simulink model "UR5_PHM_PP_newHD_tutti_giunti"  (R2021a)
settings: Solver=ode14x  StartTime=0.0  StopTime=Sim.time  FixedStep=Sim.dt  MaxStep=Sim.dt  RelTol=1e-3  EnableMultiTasking=on
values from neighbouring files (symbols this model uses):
  alpha_n = 0.98*pi/180    (= 0.0171042266695)    [parameters.m]
  alpha_t = 30*pi/180    (= 0.523598775598)    [parameters.m]
  alpha_TTS = 0    [parameters.m]
  alpha_Tw_L = -6.9e-4    (= -0.00069)    [parameters.m]
  alpha_Tw_R = 3.9e-3    (= 0.0039)    [parameters.m]
  Beta_TTS = 0    [parameters.m]
  c1 = 1e-2    (= 0.01)    [parameters.m]
  c2 = 1e-2    (= 0.01)    [parameters.m]
  c3 = 1e-2    (= 0.01)    [parameters.m]
  c4 = 1e-2    (= 0.01)    [parameters.m]
  c5 = 1e-2    (= 0.01)    [parameters.m]
  c6 = 1e-2    (= 0.01)    [parameters.m]
  Cb1 = 1.8e3    (= 1800)    [parameters.m]
  Cb2 = 1.8e3    (= 1800)    [parameters.m]
  Cb3 = 1.8e3    (= 1800)    [parameters.m]
  Cb4 = 1.8e3    (= 1800)    [parameters.m]
  Cb5 = 1.8e3    (= 1800)    [parameters.m]
  Cb6 = 1.8e3    (= 1800)    [parameters.m]
  Cth_housing = 153.90    (= 153.9)    [parameters.m]
  Cth_w = 74.20    (= 74.2)    [parameters.m]
  dt_PP = 0.05    [parameters.m]
  Fric1 = [fc_1/2 1e1 fc_1 fv_1]    [parameters.m]
  Fric2 = [fc_2/2 1e1 fc_2 fv_2]    [parameters.m]
  Fric3 = [fc_3/2 1e1 fc_3 fv_3]    [parameters.m]
  Fric4 = [fc_4/2 1e1 fc_4 fv_4]    [parameters.m]
  Fric5 = [fc_5/2 1e1 fc_5 fv_5]    [parameters.m]
  Fric6 = [fc_6/2 1e1 fc_6 fv_6]    [parameters.m]
  Hth_housing = 0.30    (= 0.3)    [parameters.m]
  Hth_w = 1.14    [parameters.m]
  I_actual = I_actual(1:10,:)    [trajcutting.m]
  J_CS1 = 7.12e-5    (= 7.12e-05)    [parameters.m]
  J_CS2 = 7.12e-5    (= 7.12e-05)    [parameters.m]
  J_CS3 = 7.12e-5    (= 7.12e-05)    [parameters.m]
  J_CS4 = 6e-6    (= 6e-06)    [parameters.m]
  J_CS5 = 6e-6    (= 6e-06)    [parameters.m]
  J_CS6 = 6e-6    (= 6e-06)    [parameters.m]
  J_FS1 = 1.62e-7    (= 1.62e-07)    [parameters.m]
  J_FS2 = 1.62e-7    (= 1.62e-07)    [parameters.m]
  J_FS3 = 1.62e-7    (= 1.62e-07)    [parameters.m]
  J_FS4 = 4.97e-8    (= 4.97e-08)    [parameters.m]
  J_FS5 = 4.97e-8    (= 4.97e-08)    [parameters.m]
  J_FS6 = 4.97e-8    (= 4.97e-08)    [parameters.m]
  J_WG1 = 3.56e-5    (= 3.56e-05)    [parameters.m]
  J_WG2 = 3.56e-5    (= 3.56e-05)    [parameters.m]
  J_WG3 = 3.56e-5    (= 3.56e-05)    [parameters.m]
  J_WG4 = 3e-6    (= 3e-06)    [parameters.m]
  J_WG5 = 3e-6    (= 3e-06)    [parameters.m]
  J_WG6 = 3e-6    (= 3e-06)    [parameters.m]
  K_i = 1    [parameters.m]
  K_p = 1    [parameters.m]
  K_torsCS1 = 4.78e6    (= 4780000)    [parameters.m]
  K_torsCS2 = 4.78e6    (= 4780000)    [parameters.m]
  K_torsCS3 = 4.78e6    (= 4780000)    [parameters.m]
  K_torsCS4 = 1.06e6    (= 1060000)    [parameters.m]
  K_torsCS5 = 1.06e6    (= 1060000)    [parameters.m]
  K_torsCS6 = 1.06e6    (= 1060000)    [parameters.m]
  K_torsWG1 = 9.56e5    (= 956000)    [parameters.m]
  K_torsWG2 = 9.56e5    (= 956000)    [parameters.m]
  K_torsWG3 = 9.56e5    (= 956000)    [parameters.m]
  K_torsWG4 = 1.84e5    (= 184000)    [parameters.m]
  K_torsWG5 = 1.84e5    (= 184000)    [parameters.m]
  K_torsWG6 = 1.84e5    (= 184000)    [parameters.m]
  K_v = 1    [parameters.m]
  Kb1 = 0.51e8    (= 51000000)    [parameters.m]
  Kb2 = 0.51e8    (= 51000000)    [parameters.m]
  Kb3 = 0.51e8    (= 51000000)    [parameters.m]
  Kb4 = 1.98e7    (= 19800000)    [parameters.m]
  Kb5 = 1.98e7    (= 19800000)    [parameters.m]
  Kb6 = 1.98e7    (= 19800000)    [parameters.m]
  Km1 = 1.2e9    (= 1200000000)    [parameters.m]
  Km2 = 1.2e9    (= 1200000000)    [parameters.m]
  Km3 = 1.2e9    (= 1200000000)    [parameters.m]
  Km4 = 5.55e8    (= 555000000)    [parameters.m]
  Km5 = 5.55e8    (= 555000000)    [parameters.m]
  Km6 = 5.55e8    (= 555000000)    [parameters.m]
  Kt1 = 0.96e5    (= 96000)    [parameters.m]
  Kt2 = 0.96e5    (= 96000)    [parameters.m]
  Kt3 = 0.96e5    (= 96000)    [parameters.m]
  Kt4 = 1.15e4    (= 11500)    [parameters.m]
  Kt5 = 1.15e4    (= 11500)    [parameters.m]
  Kt6 = 1.15e4    (= 11500)    [parameters.m]
  L = Motor.L_2/2    [parameters.m]
  m2 = polyfit(Temp(:,2),pBn_UR5_f_Temp(:,2),1)    [parameters.m]
  mb2 = polyfit(Temp(:,8),pBn_UR5_f_Temp(:,8),1)    [parameters.m]
  pickTime = t_pick(traj)    [parameters.m]
  placeTime = t_place(traj)    [parameters.m]
  q0 = q_target(1,:)    [testlaw_PP.m]
  q_CS01 = x(6)    [parameters.m]
  q_CS02 = x(6)    [parameters.m]
  q_CS03 = x(6)    [parameters.m]
  q_CS04 = x(6)    [parameters.m]
  q_CS05 = x(6)    [parameters.m]
  q_CS06 = x(6)    [parameters.m]
  q_WG01 = x(1)    [parameters.m]
  q_WG02 = x(1)    [parameters.m]
  q_WG03 = x(1)    [parameters.m]
  q_WG04 = x(1)    [parameters.m]
  q_WG05 = x(1)    [parameters.m]
  q_WG06 = x(1)    [parameters.m]
  quant_i = [Motor.imax1 Motor.imax2      Motor.imax3 Motor.imax4 Motor.imax5 Motor.imax6]/2^16    [parameters.m]
  R = Motor.R_2/2    [parameters.m]
  rg1 = 0.028    [parameters.m]
  rg2 = 0.028    [parameters.m]
  rg3 = 0.028    [parameters.m]
  rg4 = 0.0155    [parameters.m]
  rg5 = 0.0155    [parameters.m]
  rg6 = 0.0155    [parameters.m]
  sigma_p = 444.29    [parameters.m]
  sigma_v = 2*pi*1000    (= 6283.18530718)    [parameters.m]
  stiff_red = 1    [parameters.m]
  T_0 = Sim.temp    [parameters.m]
  T_switch = 1e-4    (= 0.0001)    [parameters.m]
  tau_i = 1/(fc_i*2*pi)    (= 7.95774715459e-05)    [parameters.m]
  U_s = 48    [parameters.m]
  var_i = 1e-1*[.0167 .0184 .0144 .0016      .0011 .0007]    [parameters.m]
  var_p = 1e-6*[.0943 .3877      .3478 .5436 .3400 .2081]    [parameters.m]
  var_v = 1e-4*[.0738 .1452      .1564 .4623 .1824 .0917]    [parameters.m]
  Wf_TTS_0 = 0    [parameters.m]
  Wf_TTS_ONOFF = 0    [parameters.m]
  x2_01 = x(3)    [parameters.m]
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undefined symbols (not defined in the file or in its folder): deg, Driver1, Driver2, Driver3, Driver4, Driver5, Driver6, elseif, geom, Ground, J1, J2, J3, J4, J5, J6, kg, L1, L2, L3, L4, L5, L6, LINK0, LINK1, LINK2, LINK3, LINK4, LINK5, LINK6, m, Motor, N, payload, ROBOTIQ_FT, s, Sim, Tool, X, Y, Z
libraries: sm_lib x35, nesl_utility x30, simulink x23, simulink_extras x11, spsTriangleGeneratorLib x6
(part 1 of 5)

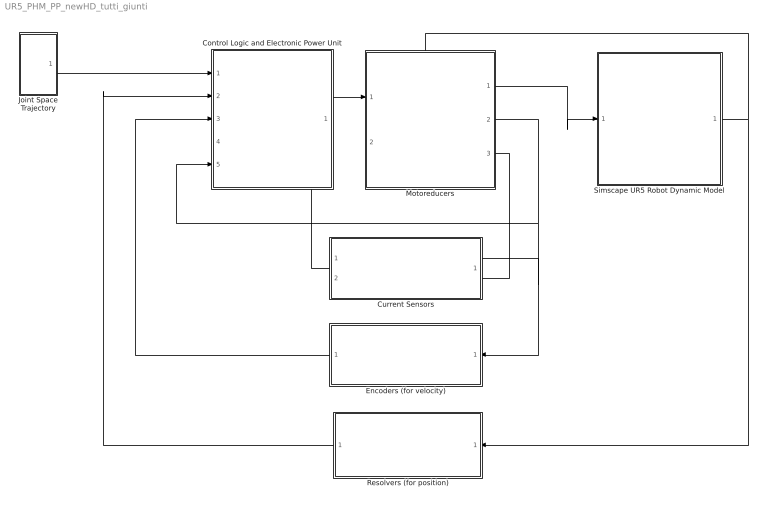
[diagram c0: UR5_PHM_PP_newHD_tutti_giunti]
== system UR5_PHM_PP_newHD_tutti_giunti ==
  Control Logic and Electronic Power Unit : Subsystem
  Current Sensors : Subsystem
  Encoders (for velocity) : Subsystem
  Joint Space Trajectory : Subsystem
  Motoreducers : Subsystem
  Resolvers (for position) : Subsystem
  Simscape UR5 Robot Dynamic Model : Subsystem
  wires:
  Resolvers (for position)/1(qFB) -> Control Logic and Electronic Power Unit/2(qFB)
  Control Logic and Electronic Power Unit/1(Vset) -> Motoreducers/1(Vset)
  Simscape UR5 Robot Dynamic Model/1(q,qd,qdd) -> Motoreducers/2(q,qd,qdd), Resolvers (for position)/1(q,qd,qdd)
  Motoreducers/1(Tu) -> Simscape UR5 Robot Dynamic Model/1(Tu)
  Joint Space Trajectory/1(qset) -> Control Logic and Electronic Power Unit/1(qset)
  Motoreducers/2(qm,qdm,qddm) -> Control Logic and Electronic Power Unit/5(qm,qdm,qddm), Current Sensors/1(qm,qdm,qddm), Encoders (for velocity)/1(qm,qdm,qddm)
  Encoders (for velocity)/1(qdmFB) -> Control Logic and Electronic Power Unit/3(qdmFB)
  Current Sensors/1(iFB) -> Control Logic and Electronic Power Unit/4(iFB)
  Motoreducers/3(i) -> Current Sensors/2(i)

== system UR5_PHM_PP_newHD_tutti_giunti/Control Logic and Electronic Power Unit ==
  qset : Inport
  qFB : Inport  Port=2
  qdmFB : Inport  Port=3
  iFB : Inport  Port=4
  qm,qdm,qddm : Inport  Port=5
  Demux{,1..3} (4 alike) : Demux  Outputs=6
  Mux : Mux  Inputs=6
  Subsystem : Subsystem
  Subsystem1 : Subsystem
  Vset : Outport
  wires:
  Demux/1 -> Subsystem/1(q1set)
  Demux/4 -> Subsystem/4(q4set)
  Demux/3 -> Subsystem/3(q3set)
  Demux1/1 -> Subsystem/7(q1FB)
  Demux/5 -> Subsystem/5(q5set)
  Demux1/2 -> Subsystem/8(q2FB)
  Demux/2 -> Subsystem/2(q2set)
  Demux/6 -> Subsystem/6(q6set)
  Demux1/3 -> Subsystem/9(q3FB)
  Demux1/5 -> Subsystem/11(q5FB)
  Demux1/6 -> Subsystem/12(q6FB)
  Subsystem/4(Vset4) -> Mux/4
  Demux1/4 -> Subsystem/10(q4FB)
  Subsystem/2(Vset2) -> Mux/2
  Subsystem/1(Vset1) -> Mux/1
  Subsystem/5(Vset5) -> Mux/5
  Subsystem/6(Vset6) -> Mux/6
  Subsystem/3(Vset3) -> Mux/3
  qFB/1 -> Demux1/1
  Mux/1 -> Vset/1
  qset/1 -> Demux/1
  Demux3/2 -> Subsystem/14(qdm2FB)
  Demux3/6 -> Subsystem/18(qdm6FB)
  Demux3/5 -> Subsystem/17(qdm5FB)
  Demux3/4 -> Subsystem/16(qdm4FB)
  Demux3/3 -> Subsystem/15(qdm3FB)
  Demux3/1 -> Subsystem/13(qdm1FB)
  qdmFB/1 -> Demux3/1
  qm,qdm,qddm/1 -> Subsystem1/1(qm,qdm,qddm)
  Subsystem1/1(qm2) -> Subsystem/25(qm2)
  Demux2/3 -> Subsystem/21(i3FB)
  Demux2/4 -> Subsystem/22(i4FB)
  Demux2/5 -> Subsystem/23(i5FB)
  Demux2/6 -> Subsystem/24(i6FB)
  Demux2/2 -> Subsystem/20(i2FB [dq0])
  Demux2/1 -> Subsystem/19(i1FB)
  iFB/1 -> Demux2/1

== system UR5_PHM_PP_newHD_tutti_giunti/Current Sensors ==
  qm,qdm,qddm : Inport
  i : Inport  Port=2
  Demux : Demux  Outputs=6
  Mux : Mux  Inputs=6
  Subsystem : Subsystem
  Subsystem1 : Subsystem
  iFB : Outport
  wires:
  Demux/1 -> Subsystem/1(i1)
  Demux/2 -> Subsystem/2(i2 [a,b,c])
  Demux/3 -> Subsystem/3(i3)
  Demux/4 -> Subsystem/4(i4)
  Demux/5 -> Subsystem/5(i5)
  Demux/6 -> Subsystem/6(i6)
  qm,qdm,qddm/1 -> Subsystem1/1(qm,qdm,qddm)
  Subsystem1/1(qm2) -> Subsystem/7(qm2)
  i/1 -> Demux/1
  Subsystem/1(i1FB) -> Mux/1
  Subsystem/2(i2FB) -> Mux/2
  Subsystem/3(i3FB) -> Mux/3
  Subsystem/4(i4FB) -> Mux/4
  Subsystem/5(i5FB) -> Mux/5
  Subsystem/6(i6FB) -> Mux/6
  Mux/1 -> iFB/1

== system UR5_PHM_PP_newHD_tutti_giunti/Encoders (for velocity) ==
  qm,qdm,qddm : Inport
  Demux1 : Demux  Outputs=6
  Mux1 : Mux  Inputs=6
  Subsystem : Subsystem
  qdmFB : Outport
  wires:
  Subsystem/1(qdm1FB) -> Mux1/1
  Demux1/4 -> Subsystem/4(qm4,qdm4,qddm4)
  Demux1/5 -> Subsystem/5(qm5,qdm5,qddm5)
  Subsystem/6(qdm6FB) -> Mux1/6
  Demux1/2 -> Subsystem/2(qm2,qdm2,qddm2)
  Subsystem/3(qdm3FB) -> Mux1/3
  Demux1/6 -> Subsystem/6(qm6,qdm6,qddm6)
  Demux1/3 -> Subsystem/3(qm3,qdm3,qddm3)
  Demux1/1 -> Subsystem/1(qm1,qdm1,qddm1)
  Subsystem/4(qdm4FB) -> Mux1/4
  Subsystem/2(qdm2FB) -> Mux1/2
  Subsystem/5(qdm5FB) -> Mux1/5
  Mux1/1 -> qdmFB/1
  qm,qdm,qddm/1 -> Demux1/1

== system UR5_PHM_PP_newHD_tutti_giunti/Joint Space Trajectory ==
  Demux{,1..5} (6 alike) : Demux  Outputs=3
  From Workspace : FromWorkspace  VariableName=qset.q1
  From Workspace1 : FromWorkspace  VariableName=qset.q2
  From Workspace2 : FromWorkspace  VariableName=qset.q3
  From Workspace3 : FromWorkspace  VariableName=qset.q4
  From Workspace4 : FromWorkspace  VariableName=qset.q5
  From Workspace5 : FromWorkspace  VariableName=qset.q6
  Mux2 : Mux  Inputs=6
  Terminator{,1..11} (12 alike) : Terminator
  qset : Outport
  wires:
  Mux2/1 -> qset/1
  Demux/2 -> Terminator/1
  Demux/3 -> Terminator1/1
  From Workspace1/1 -> Demux1/1
  Demux1/2 -> Terminator2/1
  Demux1/3 -> Terminator3/1
  Demux2/3 -> Terminator5/1
  Demux2/2 -> Terminator4/1
  From Workspace2/1 -> Demux2/1
  From Workspace3/1 -> Demux3/1
  Demux3/2 -> Terminator6/1
  Demux3/3 -> Terminator7/1
  Demux4/3 -> Terminator9/1
  Demux4/2 -> Terminator8/1
  From Workspace4/1 -> Demux4/1
  From Workspace5/1 -> Demux5/1
  Demux5/2 -> Terminator10/1
  Demux5/3 -> Terminator11/1
  From Workspace/1 -> Demux/1
  Demux/1 -> Mux2/1
  Demux1/1 -> Mux2/2
  Demux2/1 -> Mux2/3
  Demux3/1 -> Mux2/4
  Demux4/1 -> Mux2/5
  Demux5/1 -> Mux2/6

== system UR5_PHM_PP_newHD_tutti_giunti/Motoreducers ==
  Vset : Inport
  q,qd,qdd : Inport  Port=2
  Demux1 : Demux  Outputs=6
  Demux2 : Demux  Outputs=6
  Mux1 : Mux  Inputs=6
  Mux2 : Mux  Inputs=6
  Mux3 : Mux  Inputs=6
  Subsystem : Subsystem
  Tu : Outport
  qm,qdm,qddm : Outport  Port=2
  i : Outport  Port=3
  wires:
  Vset/1 -> Demux1/1
  Mux1/1 -> Tu/1
  Subsystem/5(Tu5) -> Mux1/5
  Subsystem/2(Tu2) -> Mux1/2
  Subsystem/4(Tu4) -> Mux1/4
  Demux1/1 -> Subsystem/1(Vset1)
  Demux1/3 -> Subsystem/3(Vset3)
  Demux1/6 -> Subsystem/6(Vset6)
  Subsystem/3(Tu3) -> Mux1/3
  Demux1/2 -> Subsystem/2(Vset2)
  Subsystem/6(Tu6) -> Mux1/6
  Demux1/5 -> Subsystem/5(Vset5)
  Demux1/4 -> Subsystem/4(Vset4)
  Subsystem/1(Tu1) -> Mux1/1
  Demux2/1 -> Subsystem/7(q1,qd1,qdd1)
  Demux2/2 -> Subsystem/8(q2,qd2,qdd2)
  Demux2/3 -> Subsystem/9(q3,qd3,qdd3)
  Demux2/4 -> Subsystem/10(q4,qd4,qdd4)
  Demux2/5 -> Subsystem/11(q5,qd5,qdd5)
  Demux2/6 -> Subsystem/12(q6,qd6,qdd6)
  q,qd,qdd/1 -> Demux2/1
  Subsystem/7(i1) -> Mux2/1
  Subsystem/8(i2[a,b,c]) -> Mux2/2
  Subsystem/9(i3) -> Mux2/3
  Subsystem/10(i4) -> Mux2/4
  Subsystem/11(i5) -> Mux2/5
  Subsystem/12(i6) -> Mux2/6
  Mux2/1 -> i/1
  Mux3/1 -> qm,qdm,qddm/1
  Subsystem/13(qm1,qdm1,qddm1) -> Mux3/1
  Subsystem/14(qm2,qdm2,qddm2) -> Mux3/2
  Subsystem/15(qm3,qdm3,qddm3) -> Mux3/3
  Subsystem/16(qm4,qdm4,qddm4) -> Mux3/4
  Subsystem/17(qm5,qdm5,qddm5) -> Mux3/5
  Subsystem/18(qm6,qdm6qddm6) -> Mux3/6

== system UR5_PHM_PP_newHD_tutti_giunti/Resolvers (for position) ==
  q,qd,qdd : Inport
  Demux1 : Demux  Outputs=6
  Mux1 : Mux  Inputs=6
  Subsystem : Subsystem
  qFB : Outport
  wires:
  q,qd,qdd/1 -> Demux1/1
  Mux1/1 -> qFB/1
  Subsystem/5(q5FB) -> Mux1/5
  Subsystem/2(q2FB) -> Mux1/2
  Subsystem/4(q4FB) -> Mux1/4
  Demux1/1 -> Subsystem/1(q1,qd1,qdd2)
  Demux1/3 -> Subsystem/3(q3,qd3,qdd3)
  Demux1/6 -> Subsystem/6(q6,qd6,qdd6)
  Subsystem/3(q3FB) -> Mux1/3
  Demux1/2 -> Subsystem/2(q2,qd2,qdd2)
  Subsystem/6(q6FB) -> Mux1/6
  Demux1/5 -> Subsystem/5(q5,qd5,qdd5)
  Demux1/4 -> Subsystem/4(q4,qd4,qdd4)
  Subsystem/1(q1FB) -> Mux1/1

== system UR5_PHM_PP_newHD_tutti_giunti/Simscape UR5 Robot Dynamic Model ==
  Tu : Inport
  Demux1 : Demux  Outputs=6
  Mux1 : Mux  Inputs=6
  Simscape UR5 Robot Dynamic Model1 : Subsystem
  q,qd,qdd : Outport
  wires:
  Simscape UR5 Robot Dynamic Model1/1(q1,qd1,qdd1) -> Mux1/1
  Demux1/4 -> Simscape UR5 Robot Dynamic Model1/4(T4)
  Demux1/5 -> Simscape UR5 Robot Dynamic Model1/5(T5)
  Simscape UR5 Robot Dynamic Model1/6(q6,qd6,qdd6) -> Mux1/6
  Demux1/2 -> Simscape UR5 Robot Dynamic Model1/2(T2)
  Simscape UR5 Robot Dynamic Model1/3(q3,qd3,qdd3) -> Mux1/3
  Demux1/6 -> Simscape UR5 Robot Dynamic Model1/6(T6)
  Demux1/3 -> Simscape UR5 Robot Dynamic Model1/3(T3)
  Demux1/1 -> Simscape UR5 Robot Dynamic Model1/1(T1)
  Simscape UR5 Robot Dynamic Model1/4(q4,qd4,qdd4) -> Mux1/4
  Simscape UR5 Robot Dynamic Model1/2(q2,qd2,qdd2) -> Mux1/2
  Simscape UR5 Robot Dynamic Model1/5(q5,qd5,qdd5) -> Mux1/5
  Mux1/1 -> q,qd,qdd/1
  Tu/1 -> Demux1/1

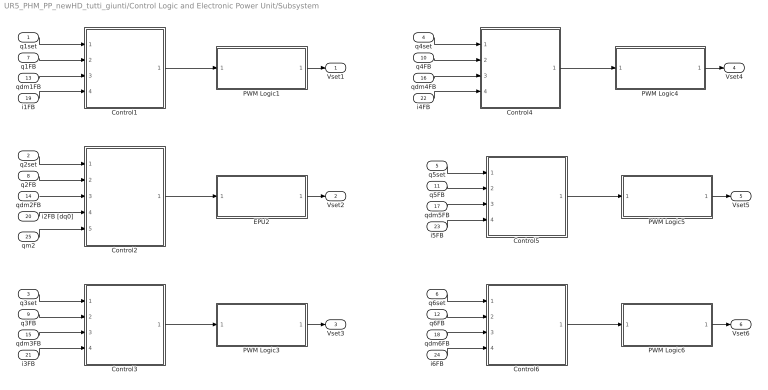
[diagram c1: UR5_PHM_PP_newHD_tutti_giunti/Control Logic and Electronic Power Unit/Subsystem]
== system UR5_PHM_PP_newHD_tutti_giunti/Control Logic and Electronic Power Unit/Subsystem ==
  q1set : Inport
  q2set : Inport  Port=2
  q3set : Inport  Port=3
  q4set : Inport  Port=4
  q5set : Inport  Port=5
  q6set : Inport  Port=6
  q1FB : Inport  Port=7
  q2FB : Inport  Port=8
  q3FB : Inport  Port=9
  q4FB : Inport  Port=10
  q5FB : Inport  Port=11
  q6FB : Inport  Port=12
  qdm1FB : Inport  Port=13
  qdm2FB : Inport  Port=14
  qdm3FB : Inport  Port=15
  qdm4FB : Inport  Port=16
  qdm5FB : Inport  Port=17
  qdm6FB : Inport  Port=18
  i1FB : Inport  Port=19
  i2FB [dq0] : Inport  Port=20
  i3FB : Inport  Port=21
  i4FB : Inport  Port=22
  i5FB : Inport  Port=23
  i6FB : Inport  Port=24
  qm2 : Inport  Port=25
  Control1 : Subsystem
  Control2 : Subsystem
  Control3 : Subsystem
  Control4 : Subsystem
  Control5 : Subsystem
  Control6 : Subsystem
  EPU2 : Subsystem
  PWM Logic1 : Subsystem
  PWM Logic3 : Subsystem
  PWM Logic4 : Subsystem
  PWM Logic5 : Subsystem
  PWM Logic6 : Subsystem
  Vset1 : Outport
  Vset2 : Outport  Port=2
  Vset3 : Outport  Port=3
  Vset4 : Outport  Port=4
  Vset5 : Outport  Port=5
  Vset6 : Outport  Port=6
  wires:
  Control5/1(V_ref) -> PWM Logic5/1(V_ref)
  qdm1FB/1 -> Control1/3(qdmFB)
  i1FB/1 -> Control1/4(iFB)
  Control1/1(V_ref) -> PWM Logic1/1(V_ref)
  PWM Logic1/1(Vset) -> Vset1/1
  Control3/1(V_ref) -> PWM Logic3/1(V_ref)
  PWM Logic3/1(Vset) -> Vset3/1
  qdm3FB/1 -> Control3/3(qdmFB)
  i3FB/1 -> Control3/4(iFB)
  PWM Logic4/1(Vset) -> Vset4/1
  Control4/1(V_ref) -> PWM Logic4/1(V_ref)
  i4FB/1 -> Control4/4(iFB)
  qdm4FB/1 -> Control4/3(qdmFB)
  PWM Logic5/1(Vset) -> Vset5/1
  qdm5FB/1 -> Control5/3(qdmFB)
  i5FB/1 -> Control5/4(iFB)
  qdm6FB/1 -> Control6/3(qdmFB)
  i6FB/1 -> Control6/4(iFB)
  Control6/1(V_ref) -> PWM Logic6/1(V_ref)
  PWM Logic6/1(Vset) -> Vset6/1
  qdm2FB/1 -> Control2/3(qdmFB)
  i2FB [dq0]/1 -> Control2/4(iFB [dq0])
  EPU2/1(Vset) -> Vset2/1
  q1set/1 -> Control1/1(qset)
  q1FB/1 -> Control1/2(qFB)
  q2set/1 -> Control2/1(qset)
  q2FB/1 -> Control2/2(qFB)
  q3set/1 -> Control3/1(qset)
  q3FB/1 -> Control3/2(qFB)
  q4set/1 -> Control4/1(qset)
  q4FB/1 -> Control4/2(qFB)
  q5set/1 -> Control5/1(qset)
  q5FB/1 -> Control5/2(qFB)
  q6set/1 -> Control6/1(qset)
  q6FB/1 -> Control6/2(qFB)
  qm2/1 -> Control2/5(qm)
  Control2/1(V[a,b,c]) -> EPU2/1(V[a,b,c])

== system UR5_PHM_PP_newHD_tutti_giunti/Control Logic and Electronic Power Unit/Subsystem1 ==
  qm,qdm,qddm : Inport
  Demux : Demux  Outputs=6
  Demux1 : Demux  Outputs=3
  Terminator{,1..6} (7 alike) : Terminator
  qm2 : Outport
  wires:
  Demux/1 -> Terminator/1
  Demux/3 -> Terminator1/1
  qm,qdm,qddm/1 -> Demux/1
  Demux/4 -> Terminator2/1
  Demux/6 -> Terminator4/1
  Demux/2 -> Demux1/1  "qm2,qdm2.qddm2"
  Demux/5 -> Terminator3/1
  Demux1/3 -> Terminator6/1
  Demux1/2 -> Terminator5/1
  Demux1/1 -> qm2/1

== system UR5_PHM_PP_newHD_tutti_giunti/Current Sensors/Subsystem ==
  i1 : Inport
  i2 [a,b,c] : Inport  Port=2
  i3 : Inport  Port=3
  i4 : Inport  Port=4
  i5 : Inport  Port=5
  i6 : Inport  Port=6
  qm2 : Inport  Port=7
  CurrentSensor1 : Subsystem
  CurrentSensor2 : Subsystem
  CurrentSensor3 : Subsystem
  CurrentSensor4 : Subsystem
  CurrentSensor5 : Subsystem
  CurrentSensor6 : Subsystem
  i1FB : Outport
  i2FB : Outport  Port=2
  i3FB : Outport  Port=3
  i4FB : Outport  Port=4
  i5FB : Outport  Port=5
  i6FB : Outport  Port=6
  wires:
  i2 [a,b,c]/1 -> CurrentSensor2/2(i2 [a,b,c])
  CurrentSensor2/1(i2 [dq0]) -> i2FB/1
  qm2/1 -> CurrentSensor2/1(qm2)
  i1/1 -> CurrentSensor1/1(i1)
  CurrentSensor1/1(i1FB) -> i1FB/1
  i3/1 -> CurrentSensor3/1(i3)
  CurrentSensor3/1(i3FB) -> i3FB/1
  i4/1 -> CurrentSensor4/1(i4)
  CurrentSensor4/1(i4FB) -> i4FB/1
  i5/1 -> CurrentSensor5/1(i5)
  CurrentSensor5/1(i5FB) -> i5FB/1
  i6/1 -> CurrentSensor6/1(i6)
  CurrentSensor6/1(i6FB) -> i6FB/1

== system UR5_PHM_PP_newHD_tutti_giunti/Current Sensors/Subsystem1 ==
  qm,qdm,qddm : Inport
  Demux : Demux  Outputs=6
  Demux1 : Demux  Outputs=3
  Terminator{,1..6} (7 alike) : Terminator
  qm2 : Outport
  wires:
  Demux/1 -> Terminator/1
  Demux/3 -> Terminator1/1
  qm,qdm,qddm/1 -> Demux/1
  Demux/4 -> Terminator2/1
  Demux/6 -> Terminator4/1
  Demux/5 -> Terminator3/1
  Demux/2 -> Demux1/1
  Demux1/1 -> qm2/1
  Demux1/2 -> Terminator5/1
  Demux1/3 -> Terminator6/1

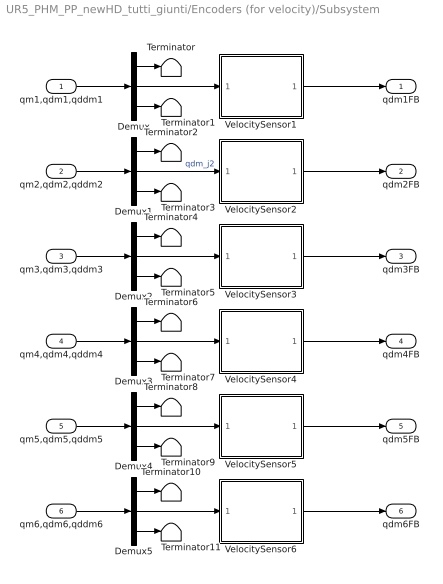
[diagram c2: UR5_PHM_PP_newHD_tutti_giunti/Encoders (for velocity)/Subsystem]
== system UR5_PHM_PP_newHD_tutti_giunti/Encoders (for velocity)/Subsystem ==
  qm1,qdm1,qddm1 : Inport
  qm2,qdm2,qddm2 : Inport  Port=2
  qm3,qdm3,qddm3 : Inport  Port=3
  qm4,qdm4,qddm4 : Inport  Port=4
  qm5,qdm5,qddm5 : Inport  Port=5
  qm6,qdm6,qddm6 : Inport  Port=6
  Demux{,1..5} (6 alike) : Demux  Outputs=3
  Terminator{,1..11} (12 alike) : Terminator
  VelocitySensor1 : Subsystem
  VelocitySensor2 : Subsystem
  VelocitySensor3 : Subsystem
  VelocitySensor4 : Subsystem
  VelocitySensor5 : Subsystem
  VelocitySensor6 : Subsystem
  qdm1FB : Outport
  qdm2FB : Outport  Port=2
  qdm3FB : Outport  Port=3
  qdm4FB : Outport  Port=4
  qdm5FB : Outport  Port=5
  qdm6FB : Outport  Port=6
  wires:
  VelocitySensor5/1(qdm5FB) -> qdm5FB/1
  VelocitySensor3/1(qdm3FB) -> qdm3FB/1
  VelocitySensor6/1(qdm6FB) -> qdm6FB/1
  VelocitySensor2/1(qdmFB2) -> qdm2FB/1
  VelocitySensor4/1(qdm4FB) -> qdm4FB/1
  Demux/3 -> Terminator1/1
  Demux/1 -> Terminator/1
  qm1,qdm1,qddm1/1 -> Demux/1
  Demux1/1 -> Terminator2/1
  Demux1/3 -> Terminator3/1
  qm2,qdm2,qddm2/1 -> Demux1/1
  Demux1/2 -> VelocitySensor2/1(qdm2)  "qdm_j2"
  Demux2/1 -> Terminator4/1
  Demux2/3 -> Terminator5/1
  qm3,qdm3,qddm3/1 -> Demux2/1
  Demux2/2 -> VelocitySensor3/1(qdm3)
  Demux3/1 -> Terminator6/1
  Demux3/3 -> Terminator7/1
  qm4,qdm4,qddm4/1 -> Demux3/1
  Demux3/2 -> VelocitySensor4/1(qdm4)
  Demux4/1 -> Terminator8/1
  Demux4/3 -> Terminator9/1
  qm5,qdm5,qddm5/1 -> Demux4/1
  Demux4/2 -> VelocitySensor5/1(qdm5)
  Demux5/1 -> Terminator10/1
  Demux5/3 -> Terminator11/1
  qm6,qdm6,qddm6/1 -> Demux5/1
  Demux5/2 -> VelocitySensor6/1(qdm6)
  Demux/2 -> VelocitySensor1/1(qdm1)
  VelocitySensor1/1(qdmFB) -> qdm1FB/1

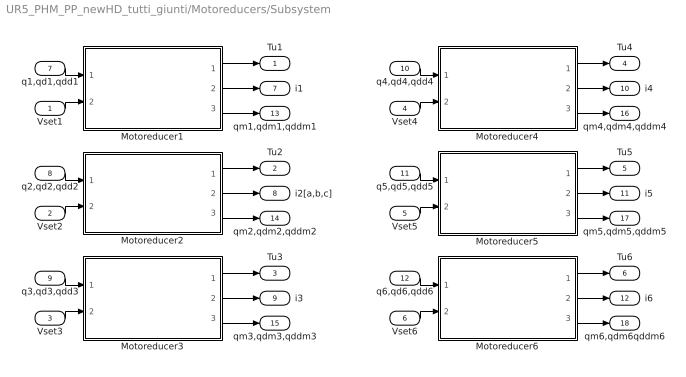
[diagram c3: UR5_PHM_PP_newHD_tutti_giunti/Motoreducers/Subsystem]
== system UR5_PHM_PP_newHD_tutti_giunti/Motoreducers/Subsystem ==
  Vset1 : Inport
  Vset2 : Inport  Port=2
  Vset3 : Inport  Port=3
  Vset4 : Inport  Port=4
  Vset5 : Inport  Port=5
  Vset6 : Inport  Port=6
  q1,qd1,qdd1 : Inport  Port=7
  q2,qd2,qdd2 : Inport  Port=8
  q3,qd3,qdd3 : Inport  Port=9
  q4,qd4,qdd4 : Inport  Port=10
  q5,qd5,qdd5 : Inport  Port=11
  q6,qd6,qdd6 : Inport  Port=12
  Motoreducer1 : Subsystem
  Motoreducer2 : Subsystem
  Motoreducer3 : Subsystem
  Motoreducer4 : Subsystem
  Motoreducer5 : Subsystem
  Motoreducer6 : Subsystem
  Tu1 : Outport
  Tu2 : Outport  Port=2
  Tu3 : Outport  Port=3
  Tu4 : Outport  Port=4
  Tu5 : Outport  Port=5
  Tu6 : Outport  Port=6
  i1 : Outport  Port=7
  i2[a,b,c] : Outport  Port=8
  i3 : Outport  Port=9
  i4 : Outport  Port=10
  i5 : Outport  Port=11
  i6 : Outport  Port=12
  qm1,qdm1,qddm1 : Outport  Port=13
  qm2,qdm2,qddm2 : Outport  Port=14
  qm3,qdm3,qddm3 : Outport  Port=15
  qm4,qdm4,qddm4 : Outport  Port=16
  qm5,qdm5,qddm5 : Outport  Port=17
  qm6,qdm6qddm6 : Outport  Port=18
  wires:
  Motoreducer5/1(Tu) -> Tu5/1
  q6,qd6,qdd6/1 -> Motoreducer6/1(q,qd,qdd)
  Vset5/1 -> Motoreducer5/2(Vset)
  q5,qd5,qdd5/1 -> Motoreducer5/1(q,qd,qdd)
  Vset1/1 -> Motoreducer1/2(Vset)
  Vset2/1 -> Motoreducer2/2(Vset)
  Vset3/1 -> Motoreducer3/2(Vset)
  q3,qd3,qdd3/1 -> Motoreducer3/1(q,qd,qdd)
  q4,qd4,qdd4/1 -> Motoreducer4/1(q,qd,qdd)
  Motoreducer4/1(Tu) -> Tu4/1
  Vset6/1 -> Motoreducer6/2(Vset)
  Vset4/1 -> Motoreducer4/2(Vset)
  Motoreducer3/1(Tu) -> Tu3/1
  q1,qd1,qdd1/1 -> Motoreducer1/1(q,qd,qdd)
  q2,qd2,qdd2/1 -> Motoreducer2/1(q,qd,qdd)
  Motoreducer6/1(Tu) -> Tu6/1
  Motoreducer2/1(Tu) -> Tu2/1
  Motoreducer1/1(Tu) -> Tu1/1
  Motoreducer1/2(i) -> i1/1
  Motoreducer2/2(i[a.b.c]) -> i2[a,b,c]/1
  Motoreducer3/2(i) -> i3/1
  Motoreducer4/2(i) -> i4/1
  Motoreducer5/2(i) -> i5/1
  Motoreducer6/2(i) -> i6/1
  Motoreducer1/3(qm,qdm,qddm) -> qm1,qdm1,qddm1/1
  Motoreducer3/3(qm,qdm,qddm) -> qm3,qdm3,qddm3/1
  Motoreducer4/3(qm,qdm,qddm) -> qm4,qdm4,qddm4/1
  Motoreducer5/3(qm,qdm,qddm) -> qm5,qdm5,qddm5/1
  Motoreducer6/3(qm,qdm,qddm) -> qm6,qdm6qddm6/1
  Motoreducer2/3(qm,qdm,qddm) -> qm2,qdm2,qddm2/1

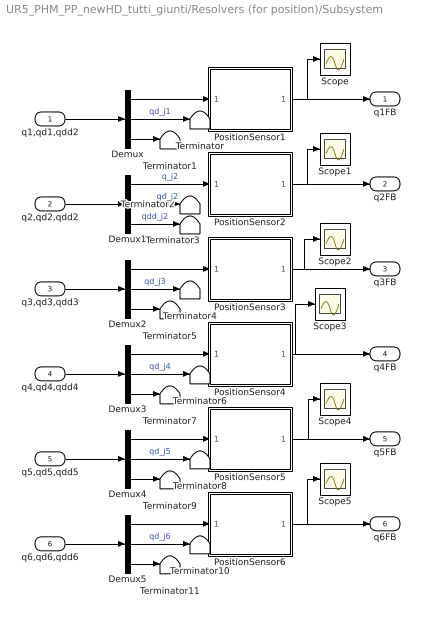
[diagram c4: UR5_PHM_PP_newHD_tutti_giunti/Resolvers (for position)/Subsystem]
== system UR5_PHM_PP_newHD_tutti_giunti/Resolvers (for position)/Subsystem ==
  q1,qd1,qdd2 : Inport
  q2,qd2,qdd2 : Inport  Port=2
  q3,qd3,qdd3 : Inport  Port=3
  q4,qd4,qdd4 : Inport  Port=4
  q5,qd5,qdd5 : Inport  Port=5
  q6,qd6,qdd6 : Inport  Port=6
  Demux{,1..5} (6 alike) : Demux  Outputs=3
  PositionSensor1 : Subsystem
  PositionSensor2 : Subsystem
  PositionSensor3 : Subsystem
  PositionSensor4 : Subsystem
  PositionSensor5 : Subsystem
  PositionSensor6 : Subsystem
  Scope{,1..5} (6 alike) : Scope
  Terminator{,1..11} (12 alike) : Terminator
  q1FB : Outport
  q2FB : Outport  Port=2
  q3FB : Outport  Port=3
  q4FB : Outport  Port=4
  q5FB : Outport  Port=5
  q6FB : Outport  Port=6
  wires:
  Demux/3 -> Terminator1/1
  Demux/1 -> PositionSensor1/1(q1)
  q1,qd1,qdd2/1 -> Demux/1
  Demux1/1 -> PositionSensor2/1(q2)  "q_j2"
  q2,qd2,qdd2/1 -> Demux1/1
  Demux1/2 -> Terminator2/1  "qd_j2"
  Demux2/3 -> Terminator5/1
  Demux2/1 -> PositionSensor3/1(q3)
  q3,qd3,qdd3/1 -> Demux2/1
  Demux2/2 -> Terminator4/1  "qd_j3"
  Demux3/3 -> Terminator7/1
  Demux3/1 -> PositionSensor4/1(q4)
  q4,qd4,qdd4/1 -> Demux3/1
  Demux3/2 -> Terminator6/1  "qd_j4"
  Demux4/3 -> Terminator9/1
  Demux4/1 -> PositionSensor5/1(q5)
  q5,qd5,qdd5/1 -> Demux4/1
  Demux4/2 -> Terminator8/1  "qd_j5"
  Demux5/3 -> Terminator11/1
  Demux5/1 -> PositionSensor6/1(q6)
  q6,qd6,qdd6/1 -> Demux5/1
  Demux5/2 -> Terminator10/1  "qd_j6"
  PositionSensor1/1(q1FB) -> Scope/1, q1FB/1
  PositionSensor2/1(q2FB) -> Scope1/1, q2FB/1
  PositionSensor3/1(q3FB) -> Scope2/1, q3FB/1
  PositionSensor4/1(q4FB) -> q4FB/1, Scope3/1
  PositionSensor5/1(q5FB) -> Scope4/1, q5FB/1
  PositionSensor6/1(q6FB) -> Scope5/1, q6FB/1
  Demux1/3 -> Terminator3/1  "qdd_j2"
  Demux/2 -> Terminator/1  "qd_j1"

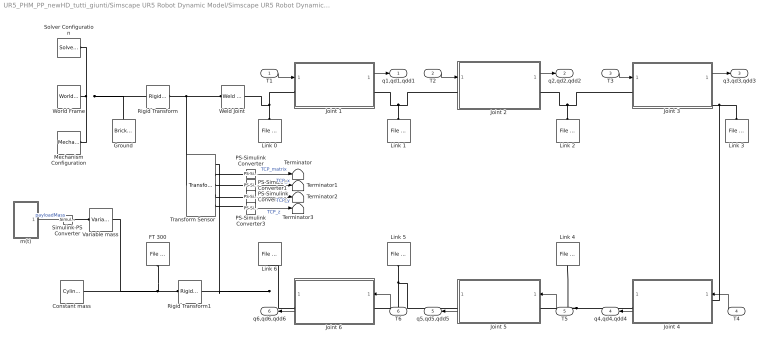
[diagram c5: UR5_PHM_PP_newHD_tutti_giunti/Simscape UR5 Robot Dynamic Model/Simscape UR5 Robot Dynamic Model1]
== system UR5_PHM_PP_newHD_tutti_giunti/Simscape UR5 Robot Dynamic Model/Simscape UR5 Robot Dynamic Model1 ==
  T1 : Inport
  T2 : Inport  Port=2
  T3 : Inport  Port=3
  T4 : Inport  Port=4
  T5 : Inport  Port=5
  T6 : Inport  Port=6
  Constant mass : sm_lib/Body Elements/Cylindrical Solid  Commented=on  GraphicAmbientColor=[0.15 0.15 0.15 1.0]  BasedOnType=Density  CenterOfMass=payload.CM  CenterOfMassUnits=m  GraphicDiffuseColor=[0.5 0.5 0.5]  CylinderLength=payload.h  CylinderLengthUnits=m  CylinderRadius=payload.r  CylinderRadiusUnits=m  Density=payload.ro  DensityUnits=kg/m^3  DoExposeReferenceFrame=on  GraphicEmissiveColor=[0.0 0.0 0.0 1.0]  ExportEntireGeometry=off  SerializedFrames=<Frames/>  MarkerShape=Sphere  MarkerSize=10  GraphicType=FromGeometry  InertiaType=Custom  Mass=payload.m  MassUnits=kg  MomentsOfInertia=payload.InertiaM  MomentsOfInertiaUnits=kg*m^2  GraphicOpacity=1.0  ProductsOfInertia=payload.InertiaP  ProductsOfInertiaUnits=kg*m^2  GraphicShininess=75  GraphicSpecularColor=[0.5 0.5 0.5 1.0]  GraphicVisPropType=SimpleVisualProperties
  FT 300 : sm_lib/Body Elements/File Solid  Commented=on  ExtGeomFileName=geom\ROBOTIQ_FT-300.STEP  UnitType=Custom  ExtGeomFileUnits=mm  StepReaderType=HEX  ExportConvexHullGeometry=off  InertiaType=Custom  Mass=Tool.Mass  MassUnits=kg  CenterOfMass=Tool.CM  CenterOfMassUnits=m  MomentsOfInertia=Tool.InertiaM  MomentsOfInertiaUnits=kg*m^2  ProductsOfInertia=Tool.InertiaP  ProductsOfInertiaUnits=kg*m^2  BasedOnType=DensityFromFile  Density=1000  DensityUnits=kg/m^3  DoExposeReferenceFrame=on  SerializedFrames=<Frames/>  GraphicType=FromGeometry  MarkerShape=Sphere  MarkerSize=10  GraphicVisPropType=SimpleVisualProperties  GraphicDiffuseColor=[0.0 0.0 0.0]  GraphicSpecularColor=[0.5 0.5 0.5 1.0]  GraphicAmbientColor=[0.15 0.15 0.15 1.0]  GraphicEmissiveColor=[0.0 0.0 0.0 1.0]  GraphicShininess=75  GraphicOpacity=1.0
  Ground : sm_lib/Body Elements/Brick Solid  GraphicAmbientColor=[0.15 0.15 0.15 1.0]  BasedOnType=Density  BrickDimensions=[Ground.l Ground.w Ground.h]  BrickDimensionUnits=m  CenterOfMass=[0 0 0]  CenterOfMassUnits=m  GraphicDiffuseColor=[0.5 0.5 0.5]  Density=1000  DensityUnits=kg/m^3  DoExposeReferenceFrame=on  GraphicEmissiveColor=[0.0 0.0 0.0 1.0]  ExportEntireGeometry=off  SerializedFrames=<Frames/>  MarkerShape=Sphere  MarkerSize=10  GraphicType=FromGeometry  InertiaType=CalculateFromGeometry  Mass=1  MassUnits=kg  MomentsOfInertia=[1 1 1]  MomentsOfInertiaUnits=kg*m^2  GraphicOpacity=1.0  ProductsOfInertia=[0 0 0]  ProductsOfInertiaUnits=kg*m^2  GraphicShininess=75  GraphicSpecularColor=[0.5 0.5 0.5 1.0]  GraphicVisPropType=SimpleVisualProperties
  Joint 1 : Subsystem
  Joint 2 : Subsystem
  Joint 3 : Subsystem
  Joint 4 : Subsystem
  Joint 5 : Subsystem
  Joint 6 : Subsystem
  Link 0 : sm_lib/Body Elements/File Solid  ExtGeomFileName=geom\LINK0.STEP  UnitType=Custom  ExtGeomFileUnits=mm  StepReaderType=HEX  ExportConvexHullGeometry=off  InertiaType=Custom  Mass=1  MassUnits=kg  CenterOfMass=[0 0 0]  CenterOfMassUnits=m  MomentsOfInertia=[1 1 1]  MomentsOfInertiaUnits=kg*m^2  ProductsOfInertia=[0 0 0]  ProductsOfInertiaUnits=kg*m^2  BasedOnType=DensityFromFile  Density=1000  DensityUnits=kg/m^3  DoExposeReferenceFrame=on  SerializedFrames=<Frames/>  GraphicType=FromGeometry  MarkerShape=Sphere  MarkerSize=10  GraphicVisPropType=SimpleVisualProperties  GraphicDiffuseColor=[0.8 0.8 1.0]  GraphicSpecularColor=[0.5 0.5 0.5 1.0]  GraphicAmbientColor=[0.15 0.15 0.15 1.0]  GraphicEmissiveColor=[0.0 0.0 0.0 1.0]  GraphicShininess=75  GraphicOpacity=1.0
  Link 1 : sm_lib/Body Elements/File Solid  ExtGeomFileName=geom\LINK1.STEP  UnitType=Custom  ExtGeomFileUnits=mm  StepReaderType=HEX  ExportConvexHullGeometry=off  InertiaType=Custom  Mass=L1.Mass  MassUnits=kg  CenterOfMass=L1.CM  CenterOfMassUnits=m  MomentsOfInertia=L1.InertiaM  MomentsOfInertiaUnits=kg*m^2  ProductsOfInertia=L1.InertiaP  ProductsOfInertiaUnits=kg*m^2  BasedOnType=DensityFromFile  Density=1000  DensityUnits=kg/m^3  DoExposeReferenceFrame=on  SerializedFrames=<Frames/>  GraphicType=FromGeometry  MarkerShape=Sphere  MarkerSize=10  GraphicVisPropType=SimpleVisualProperties  GraphicDiffuseColor=[0.8 0.8 1.0]  GraphicSpecularColor=[0.5 0.5 0.5 1.0]  GraphicAmbientColor=[0.15 0.15 0.15 1.0]  GraphicEmissiveColor=[0.0 0.0 0.0 1.0]  GraphicShininess=75  GraphicOpacity=1.0
  Link 2 : sm_lib/Body Elements/File Solid  ExtGeomFileName=geom\LINK2.STEP  UnitType=Custom  ExtGeomFileUnits=mm  StepReaderType=HEX  ExportConvexHullGeometry=off  InertiaType=Custom  Mass=L2.Mass  MassUnits=kg  CenterOfMass=L2.CM  CenterOfMassUnits=m  MomentsOfInertia=L2.InertiaM  MomentsOfInertiaUnits=kg*m^2  ProductsOfInertia=L2.InertiaP  ProductsOfInertiaUnits=kg*m^2  BasedOnType=DensityFromFile  Density=1000  DensityUnits=kg/m^3  DoExposeReferenceFrame=on  SerializedFrames=<Frames/>  GraphicType=FromGeometry  MarkerShape=Sphere  MarkerSize=10  GraphicVisPropType=SimpleVisualProperties  GraphicDiffuseColor=[0.8 0.8 1.0]  GraphicSpecularColor=[0.5 0.5 0.5 1.0]  GraphicAmbientColor=[0.15 0.15 0.15 1.0]  GraphicEmissiveColor=[0.0 0.0 0.0 1.0]  GraphicShininess=75  GraphicOpacity=1.0
  Link 3 : sm_lib/Body Elements/File Solid  ExtGeomFileName=geom\LINK3.STEP  UnitType=Custom  ExtGeomFileUnits=mm  StepReaderType=HEX  ExportConvexHullGeometry=off  InertiaType=Custom  Mass=L3.Mass  MassUnits=kg  CenterOfMass=L3.CM  CenterOfMassUnits=m  MomentsOfInertia=L3.InertiaM  MomentsOfInertiaUnits=kg*m^2  ProductsOfInertia=L3.InertiaP  ProductsOfInertiaUnits=kg*m^2  BasedOnType=DensityFromFile  Density=1000  DensityUnits=kg/m^3  DoExposeReferenceFrame=on  SerializedFrames=<Frames/>  GraphicType=FromGeometry  MarkerShape=Sphere  MarkerSize=10  GraphicVisPropType=SimpleVisualProperties  GraphicDiffuseColor=[0.8 0.8 1.0]  GraphicSpecularColor=[0.5 0.5 0.5 1.0]  GraphicAmbientColor=[0.15 0.15 0.15 1.0]  GraphicEmissiveColor=[0.0 0.0 0.0 1.0]  GraphicShininess=75  GraphicOpacity=1.0
  Link 4 : sm_lib/Body Elements/File Solid  ExtGeomFileName=geom\LINK4.STEP  UnitType=Custom  ExtGeomFileUnits=mm  StepReaderType=HEX  ExportConvexHullGeometry=off  InertiaType=Custom  Mass=L4.Mass  MassUnits=kg  CenterOfMass=L4.CM  CenterOfMassUnits=m  MomentsOfInertia=L4.InertiaM  MomentsOfInertiaUnits=kg*m^2  ProductsOfInertia=L4.InertiaP  ProductsOfInertiaUnits=kg*m^2  BasedOnType=DensityFromFile  Density=1000  DensityUnits=kg/m^3  DoExposeReferenceFrame=on  SerializedFrames=<Frames/>  GraphicType=FromGeometry  MarkerShape=Sphere  MarkerSize=10  GraphicVisPropType=SimpleVisualProperties  GraphicDiffuseColor=[0.8 0.8 1.0]  GraphicSpecularColor=[0.5 0.5 0.5 1.0]  GraphicAmbientColor=[0.15 0.15 0.15 1.0]  GraphicEmissiveColor=[0.0 0.0 0.0 1.0]  GraphicShininess=75  GraphicOpacity=1.0
  Link 5 : sm_lib/Body Elements/File Solid  ExtGeomFileName=geom\LINK5.STEP  UnitType=Custom  ExtGeomFileUnits=mm  StepReaderType=HEX  ExportConvexHullGeometry=off  InertiaType=Custom  Mass=L5.Mass  MassUnits=kg  CenterOfMass=L5.CM  CenterOfMassUnits=m  MomentsOfInertia=L5.InertiaM  MomentsOfInertiaUnits=kg*m^2  ProductsOfInertia=L5.InertiaP  ProductsOfInertiaUnits=kg*m^2  BasedOnType=DensityFromFile  Density=1000  DensityUnits=kg/m^3  DoExposeReferenceFrame=on  SerializedFrames=<Frames/>  GraphicType=FromGeometry  MarkerShape=Sphere  MarkerSize=10  GraphicVisPropType=SimpleVisualProperties  GraphicDiffuseColor=[0.8 0.8 1.0]  GraphicSpecularColor=[0.5 0.5 0.5 1.0]  GraphicAmbientColor=[0.15 0.15 0.15 1.0]  GraphicEmissiveColor=[0.0 0.0 0.0 1.0]  GraphicShininess=75  GraphicOpacity=1.0
  Link 6 : sm_lib/Body Elements/File Solid  ExtGeomFileName=geom\LINK6.STEP  UnitType=Custom  ExtGeomFileUnits=mm  StepReaderType=HEX  ExportConvexHullGeometry=off  InertiaType=Custom  Mass=L6.Mass  MassUnits=kg  CenterOfMass=L6.CM  CenterOfMassUnits=m  MomentsOfInertia=L6.InertiaM  MomentsOfInertiaUnits=kg*m^2  ProductsOfInertia=L6.InertiaP  ProductsOfInertiaUnits=kg*m^2  BasedOnType=DensityFromFile  Density=1000  DensityUnits=kg/m^3  DoExposeReferenceFrame=on  SerializedFrames=<Frames/>  GraphicType=FromGeometry  MarkerShape=Sphere  MarkerSize=10  GraphicVisPropType=SimpleVisualProperties  GraphicDiffuseColor=[0.8 0.8 1.0]  GraphicSpecularColor=[0.5 0.5 0.5 1.0]  GraphicAmbientColor=[0.15 0.15 0.15 1.0]  GraphicEmissiveColor=[0.0 0.0 0.0 1.0]  GraphicShininess=75  GraphicOpacity=1.0
  Mechanism Configuration : sm_lib/Utilities/Mechanism Configuration  UniformGravity=Constant  GravityVector=[0 0 -9.80665]  GravityVectorUnits=m/s^2  GravityUnits=m/s^2  LinearizationDelta=0.001  JointModeTransitionNonlinearIterations=2
  PS-Simulink Converter{,1..3} (4 alike) : nesl_utility/PS-Simulink Converter  PhysicalDomain=network_engine_domain  SubClassName=ps_output  LeftPortType=input  RightPortType=output  PseudoPeriodic=off  Frequencies=[]  Unit=inherit  AffineConversion=off
  Rigid Transform : sm_lib/Frames and Transforms/Rigid Transform  TranslationMethod=Cartesian  TranslationStandardOffset=0  TranslationLengthUnit=m  TranslationStandardAxis=+Z  TranslationCartesianOffset=[0 0 Ground.h/2]  TranslationROffset=0  TranslationROffsetUnits=m  TranslationZOffset=0  TranslationZOffsetUnits=m  TranslationThetaOffset=0  TranslationThetaOffsetUnits=deg  RotationMethod=None  RotationAngleUnits=deg  RotationStandardAxis=+Z  RotationAngle=0.0  RotationArbitraryAxis=[0 0 1]  FollAlignAxisA=+X  BaseAlignAxisA=+Y  FollAlignAxisB=+Y  BaseAlignAxisB=+Z  RotationSequenceAxes=FollowerAxes  RotationSequence=XYX  RotationSequenceAngles=[0 0 0]  RotationSequenceAnglesUnits=deg  RotationMatrix=[1 0 0; 0 1 0; 0 0 1]
  Rigid Transform1 : sm_lib/Frames and Transforms/Rigid Transform  TranslationMethod=Cartesian  TranslationStandardOffset=0  TranslationLengthUnit=m  TranslationStandardAxis=+Z  TranslationCartesianOffset=[0 0 0]  TranslationROffset=0  TranslationROffsetUnits=m  TranslationZOffset=0  TranslationZOffsetUnits=m  TranslationThetaOffset=0  TranslationThetaOffsetUnits=deg  RotationMethod=AlignedAxes  RotationAngleUnits=deg  RotationStandardAxis=+Z  RotationAngle=0.0  RotationArbitraryAxis=[0 0 1]  FollAlignAxisA=+Z  BaseAlignAxisA=-Z  FollAlignAxisB=+Y  BaseAlignAxisB=+Y  RotationSequenceAxes=FollowerAxes  RotationSequence=XYX  RotationSequenceAngles=[0 0 0]  RotationSequenceAnglesUnits=deg  RotationMatrix=[1 0 0; 0 1 0; 0 0 1]
  Simulink-PS Converter : nesl_utility/Simulink-PS Converter  PhysicalDomain=network_engine_domain  SubClassName=ps_input  LeftPortType=input  RightPortType=output  PseudoPeriodic=off  Frequencies=[]  NoiseDistribution=none  NoiseParameters=[]  Unit=1  AffineConversion=off  FilteringAndDerivatives=provide  SimscapeFilterOrder=1  InputFilterTimeConstant=0.001  UdotUserProvided=0
  Solver Configuration : nesl_utility/Solver Configuration  PhysicalDomain=network_engine_domain  SubClassName=solver  LeftPortType=input  RightPortType=generic  Tones=[]  Harmonics=[]  SimulateNoise=off  Profile=off  UseLocalSampling=off  EnableSwitchedLinearOptims=on  FrequencyDomain=off  UseCCode=off  RelTol=0.001  AbsTol=1e-06  MinStep=1e-09  ToWorkspace=off  RevertToSquareIcSolve=off  NumHomotopyIterations=100  PhasorMode=off  PhasorModeNumHarmonics=1  DoDC=off  ResidualTolerance=1e-09  UseLocalSolver=off  LocalSolverChoice=NE_BACKWARD_EULER_ADVANCER  LocalSolverSampleTime=0.001  DoFixedCost=off  MaxNonlinIter=3  MaxModeIter=2  ComputeImpulses=off  ImpulseIterations=2  LinearAlgebra=Full  EquationFormulation=NE_TIME_EF  DelaysMemoryBudget=1024  AutomaticFiltering=on  FilteringTimeConstant=0.001  PartitionStorageMethod=AS_NEEDED  PartitionMemoryBudget=1024  PartitionMethod=FAST
  Terminator{,1..3} (4 alike) : Terminator
  Transform Sensor : sm_lib/Frames and Transforms/Transform Sensor  MeasurementFrame=World  SenseAngle=off  SenseAxis=off  SenseAngle1=off  SenseAngle2=off  SenseAngle3=off  SenseQ=off  SenseR=on  SenseOmegaX=off  SenseOmegaY=off  SenseOmegaZ=off  SenseOmega1=off  SenseOmega2=off  SenseOmega3=off  SenseQDot=off  SenseRDot=off  SenseAlphaX=off  SenseAlphaY=off  SenseAlphaZ=off  SenseAlpha1=off  SenseAlpha2=off  SenseAlpha3=off  SenseQDDot=off  SenseRDDot=off  SenseX=on  SenseY=on  SenseZ=on  SenseRad=off  SenseAzim=off  SenseDist=off  SenseInc=off  SenseXDot=off  SenseYDot=off  SenseZDot=off  SenseRadDot=off  SenseAzimDot=off  SenseDistDot=off  SenseIncDot=off  SenseXDDot=off  SenseYDDot=off  SenseZDDot=off  SenseRadDDot=off  SenseAzimDDot=off  SenseDistDDot=off  SenseIncDDot=off
  Variable mass : sm_lib/Body Elements/Variable Mass/Variable Cylindrical Solid  LengthType=Constant  Length=payload.h  LengthUnits=m  RadiusType=Constant  Radius=payload.r  RadiusUnits=m  MassType=ProvidedByInput  InitialMassType=Specified  InitialMass=1  InitialMassUnits=kg  Density=1000  DensityUnits=kg/m^3  SenseRadius=off  SenseLength=off  SenseMass=off  SenseCenterOfMass=off  SenseInertiaMatrix=off  GraphicType=FromGeometry  MarkerShape=Sphere  MarkerSize=10  GraphicVisPropType=SimpleVisualProperties  GraphicDiffuseColor=[0.5 0.5 0.5]  GraphicSpecularColor=[0.5 0.5 0.5 1.0]  GraphicAmbientColor=[0.15 0.15 0.15 1.0]  GraphicEmissiveColor=[0.0 0.0 0.0 1.0]  GraphicShininess=75  GraphicOpacity=1.0
  Weld Joint : sm_lib/Joints/Weld Joint  JointMode=Normal  SenseConstraintForce=off  SenseConstraintForceX=off  SenseConstraintForceY=off  SenseConstraintForceZ=off  SenseConstraintTorque=off  SenseConstraintTorqueX=off  SenseConstraintTorqueY=off  SenseConstraintTorqueZ=off  SenseTotalForce=off  SenseTotalForceX=off  SenseTotalForceY=off  SenseTotalForceZ=off  SenseTotalTorque=off  SenseTotalTorqueX=off  SenseTotalTorqueY=off  SenseTotalTorqueZ=off  CompositeWrenchDir=FollowerOnBase  CompositeWrenchFrame=BaseFrame
  World Frame : sm_lib/Frames and Transforms/World Frame
  m(t) : Subsystem
  q1,qd1,qdd1 : Outport
  q2,qd2,qdd2 : Outport  Port=2
  q3,qd3,qdd3 : Outport  Port=3
  q4,qd4,qdd4 : Outport  Port=4
  q5,qd5,qdd5 : Outport  Port=5
  q6,qd6,qdd6 : Outport  Port=6
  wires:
  T1/1 -> Joint 1/1(T1)
  Joint 1/1(q1,qd1,qdd1) -> q1,qd1,qdd1/1
  T2/1 -> Joint 2/1(T2)
  Joint 2/1(q2,qd2,qdd2) -> q2,qd2,qdd2/1
  Joint 3/1(q3,qd3,qdd3) -> q3,qd3,qdd3/1
  Joint 4/1(q4,qd4,qdd4) -> q4,qd4,qdd4/1
  Joint 5/1(q5,qd5,qdd5) -> q5,qd5,qdd5/1
  Joint 6/1(q6,qd6,qdd6) -> q6,qd6,qdd6/1
  T3/1 -> Joint 3/1(T3)
  T4/1 -> Joint 4/1(T4)
  T5/1 -> Joint 5/1(T5)
  T6/1 -> Joint 6/1(T6)
  PS-Simulink Converter/1 -> Terminator/1  "TCP_matrix"
  PS-Simulink Converter1/1 -> Terminator1/1  "TCP_x"
  PS-Simulink Converter2/1 -> Terminator2/1  "TCP_y"
  PS-Simulink Converter3/1 -> Terminator3/1  "TCP_z"
  m(t)/1(Out1) -> Simulink-PS Converter/1  "payloadMass"
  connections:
  Weld Joint/LConn1 -- Transform Sensor/LConn1 -- Rigid Transform/RConn1
  Joint 4/RConn1 -- Link 4/RConn1 -- Joint 5/LConn1
  Link 2/RConn1 -- Joint 2/RConn1 -- Joint 3/LConn1
  Link 1/RConn1 -- Joint 1/RConn1 -- Joint 2/LConn1
  Link 3/RConn1 -- Joint 3/RConn1 -- Joint 4/LConn1
  Mechanism Configuration/RConn1 -- Rigid Transform/LConn1 -- Ground/RConn1 -- World Frame/RConn1 -- Solver Configuration/RConn1
  Joint 6/RConn1 -- Transform Sensor/RConn1 -- Rigid Transform1/LConn1 -- Link 6/RConn1
  Link 5/RConn1 -- Joint 5/RConn1 -- Joint 6/LConn1
  Link 0/RConn1 -- Weld Joint/RConn1 -- Joint 1/LConn1
  FT 300/RConn1 -- Variable mass/RConn1 -- Constant mass/RConn1 -- Rigid Transform1/RConn1
  Transform Sensor/RConn2 -- PS-Simulink Converter/LConn1
  Transform Sensor/RConn3 -- PS-Simulink Converter1/LConn1
  Transform Sensor/RConn4 -- PS-Simulink Converter2/LConn1
  PS-Simulink Converter3/LConn1 -- Transform Sensor/RConn5
  Simulink-PS Converter/RConn1 -- Variable mass/LConn1

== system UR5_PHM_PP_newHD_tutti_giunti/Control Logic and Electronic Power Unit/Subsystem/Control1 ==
  qset : Inport
  qFB : Inport  Port=2
  qdmFB : Inport  Port=3
  iFB : Inport  Port=4
  P Position Controller : Subsystem
  PI Current Controller : Subsystem
  PI Velocity Controller : Subsystem
  Sum : Sum  Inputs=|+-
  Sum1 : Sum  Inputs=|+-
  Sum2 : Sum  Inputs=|+-
  V_ref : Outport
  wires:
  qset/1 -> Sum/1  "qSet_j1"
  Sum/1 -> P Position Controller/1(q_error)
  Sum2/1 -> PI Current Controller/1(i_error)
  PI Current Controller/1(V_ref) -> V_ref/1
  P Position Controller/1(qdm_ref) -> Sum1/1  "qdmRef_j1"
  qFB/1 -> Sum/2  "qFB_j1"
  iFB/1 -> Sum2/2  "iFB_j1"
  Sum1/1 -> PI Velocity Controller/1(qdm_error)
  qdmFB/1 -> Sum1/2  "qdmFB_j1"
  PI Velocity Controller/1(i_ref) -> Sum2/1  "iRef_j1"

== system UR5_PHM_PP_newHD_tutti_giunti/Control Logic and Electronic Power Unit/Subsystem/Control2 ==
  qset : Inport
  qFB : Inport  Port=2
  qdmFB : Inport  Port=3
  iFB [dq0] : Inport  Port=4
  qm : Inport  Port=5
  Current Controller : Subsystem
  Inverse Park Transformation : Subsystem
  P Position Controller : Subsystem
  PI Velocity Controller : Subsystem
  Sum : Sum  Inputs=|+-
  Sum1 : Sum  Inputs=|+-
  V[a,b,c] : Outport
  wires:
  iFB [dq0]/1 -> Current Controller/2(i_FB [dq0])
  qdmFB/1 -> Sum1/2  "qdmFB_j2"
  qFB/1 -> Sum/2  "qFB_j2"
  Current Controller/1(V[d,q,0]) -> Inverse Park Transformation/1(V[d,q,0])  "V[d,q,0]"
  Sum/1 -> P Position Controller/1(q_error)
  Sum1/1 -> PI Velocity Controller/1(qdm_error)
  Inverse Park Transformation/1(V[a,b,c]) -> V[a,b,c]/1  "V[a,b,c]"
  qm/1 -> Inverse Park Transformation/2(qm)
  P Position Controller/1(qdm_ref) -> Sum1/1  "qdmRef_j2"
  qset/1 -> Sum/1  "qSet_j2"
  PI Velocity Controller/1(i_ref) -> Current Controller/1(i_ref)  "iRef_j2"

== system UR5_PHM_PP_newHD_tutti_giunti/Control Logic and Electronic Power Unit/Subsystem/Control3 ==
  qset : Inport
  qFB : Inport  Port=2
  qdmFB : Inport  Port=3
  iFB : Inport  Port=4
  P Position Controller : Subsystem
  PI Current Controller : Subsystem
  PI Velocity Controller : Subsystem
  Sum : Sum  Inputs=|+-
  Sum1 : Sum  Inputs=|+-
  Sum2 : Sum  Inputs=|+-
  V_ref : Outport
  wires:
  Sum2/1 -> PI Current Controller/1(i_error)
  Sum/1 -> P Position Controller/1(q_error)
  P Position Controller/1(qdm_ref) -> Sum1/1  "qdmRef_j3"
  PI Current Controller/1(V_ref) -> V_ref/1
  iFB/1 -> Sum2/2  "iFB_j3"
  qdmFB/1 -> Sum1/2  "qdmFB_j3"
  Sum1/1 -> PI Velocity Controller/1(qdm_error)
  qFB/1 -> Sum/2  "qFB_j3"
  qset/1 -> Sum/1  "qSet_j3"
  PI Velocity Controller/1(i_ref) -> Sum2/1  "iRef_j3"

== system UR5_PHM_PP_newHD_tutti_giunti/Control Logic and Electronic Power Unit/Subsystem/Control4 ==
  qset : Inport
  qFB : Inport  Port=2
  qdmFB : Inport  Port=3
  iFB : Inport  Port=4
  P Position Controller : Subsystem
  PI Current Controller : Subsystem
  PI Velocity Controller : Subsystem
  Sum : Sum  Inputs=|+-
  Sum1 : Sum  Inputs=|+-
  Sum2 : Sum  Inputs=|+-
  V_ref : Outport
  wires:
  P Position Controller/1(qdm_ref) -> Sum1/1  "qdmRef_j4"
  PI Current Controller/1(V_ref) -> V_ref/1
  Sum2/1 -> PI Current Controller/1(i_error)
  Sum1/1 -> PI Velocity Controller/1(qdm_error)
  Sum/1 -> P Position Controller/1(q_error)
  qFB/1 -> Sum/2  "qFB_j4"
  qdmFB/1 -> Sum1/2  "qdmFB_j4"
  iFB/1 -> Sum2/2  "iFB_j4"
  qset/1 -> Sum/1  "qSet_j4"
  PI Velocity Controller/1(i_ref) -> Sum2/1  "iRef_j4"

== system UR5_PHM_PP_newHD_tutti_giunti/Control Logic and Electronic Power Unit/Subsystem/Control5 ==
  qset : Inport
  qFB : Inport  Port=2
  qdmFB : Inport  Port=3
  iFB : Inport  Port=4
  P Position Controller : Subsystem
  PI Current Controller : Subsystem
  PI Velocity Controller : Subsystem
  Sum : Sum  Inputs=|+-
  Sum1 : Sum  Inputs=|+-
  Sum2 : Sum  Inputs=|+-
  V_ref : Outport
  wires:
  iFB/1 -> Sum2/2  "iFB_j5"
  P Position Controller/1(qdm_ref) -> Sum1/1  "qdmRef_j5"
  Sum/1 -> P Position Controller/1(q_error)
  Sum2/1 -> PI Current Controller/1(i_error)
  PI Current Controller/1(V_ref) -> V_ref/1
  qFB/1 -> Sum/2  "qFB_j5"
  Sum1/1 -> PI Velocity Controller/1(qdm_error)
  qdmFB/1 -> Sum1/2  "qdmFB_j5"
  qset/1 -> Sum/1  "qSet_j5"
  PI Velocity Controller/1(i_ref) -> Sum2/1  "iRef_j5"

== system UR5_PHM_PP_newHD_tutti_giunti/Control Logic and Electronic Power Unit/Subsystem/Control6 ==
  qset : Inport
  qFB : Inport  Port=2
  qdmFB : Inport  Port=3
  iFB : Inport  Port=4
  P Position Controller : Subsystem
  PI Current Controller : Subsystem
  PI Velocity Controller : Subsystem
  Sum : Sum  Inputs=|+-
  Sum1 : Sum  Inputs=|+-
  Sum2 : Sum  Inputs=|+-
  V_ref : Outport
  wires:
  Sum/1 -> P Position Controller/1(q_error)
  P Position Controller/1(qdm_ref) -> Sum1/1  "qdmRef_j6"
  iFB/1 -> Sum2/2  "iFB_j6"
  qFB/1 -> Sum/2  "qFB_j6"
  PI Current Controller/1(V_ref) -> V_ref/1
  Sum1/1 -> PI Velocity Controller/1(qdm_error)
  qdmFB/1 -> Sum1/2  "qdmFB_j6"
  Sum2/1 -> PI Current Controller/1(i_error)
  qset/1 -> Sum/1  "qSet_j6"
  PI Velocity Controller/1(i_ref) -> Sum2/1  "iRef_j6"

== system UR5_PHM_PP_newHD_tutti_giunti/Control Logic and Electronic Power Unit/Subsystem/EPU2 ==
  V[a,b,c] : Inport
  Inverter : Subsystem
  PWM : Subsystem
  Supply voltage : Constant  Value=U_s
  Vset : Outport
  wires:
  Supply voltage/1 -> Inverter/2(V_dclink), PWM/2(V_dclink)
  PWM/1(q[a,b,c]) -> Inverter/1(q[a,b,c])
  Inverter/1(V[ao,bo,co]) -> Vset/1
  V[a,b,c]/1 -> PWM/1(V*[a,b,c])

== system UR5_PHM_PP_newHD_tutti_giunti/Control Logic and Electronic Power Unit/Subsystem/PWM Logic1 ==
  V_ref : Inport
  PWM Modulator : Subsystem
  Scope : Scope
  Simplified inverter : Subsystem
  Supply voltage : Constant  Value=U_s
  Vset : Outport
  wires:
  PWM Modulator/2(q2) -> Simplified inverter/3(q2)
  PWM Modulator/1(q1) -> Simplified inverter/2(q1)
  V_ref/1 -> PWM Modulator/2(V_ref)
  Simplified inverter/1(Vset) -> Scope/1, Vset/1
  Supply voltage/1 -> Simplified inverter/1(Supply voltage), PWM Modulator/1(Supply voltage)

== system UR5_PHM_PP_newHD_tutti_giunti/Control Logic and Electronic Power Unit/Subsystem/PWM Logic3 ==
  V_ref : Inport
  PWM Modulator : Subsystem
  Simplified inverter : Subsystem
  Supply voltage : Constant  Value=U_s
  Vset : Outport
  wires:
  PWM Modulator/2(q2) -> Simplified inverter/3(q2)
  PWM Modulator/1(q1) -> Simplified inverter/2(q1)
  V_ref/1 -> PWM Modulator/2(Compensated error)
  Simplified inverter/1(Vset) -> Vset/1
  Supply voltage/1 -> Simplified inverter/1(Supply voltage), PWM Modulator/1(Supply voltage)

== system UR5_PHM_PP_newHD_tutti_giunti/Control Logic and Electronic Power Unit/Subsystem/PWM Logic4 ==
  V_ref : Inport
  PWM Modulator : Subsystem
  Simplified inverter : Subsystem
  Supply voltage : Constant  Value=U_s
  Vset : Outport
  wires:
  Supply voltage/1 -> PWM Modulator/1(Supply voltage), Simplified inverter/1(Supply voltage)
  Simplified inverter/1(Vset) -> Vset/1
  V_ref/1 -> PWM Modulator/2(Compensated error)
  PWM Modulator/1(q1) -> Simplified inverter/2(q1)
  PWM Modulator/2(q2) -> Simplified inverter/3(q2)

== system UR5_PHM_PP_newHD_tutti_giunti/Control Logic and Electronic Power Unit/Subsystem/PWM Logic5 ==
  V_ref : Inport
  PWM Modulator : Subsystem
  Simplified inverter : Subsystem
  Supply voltage : Constant  Value=U_s
  Vset : Outport
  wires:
  PWM Modulator/2(q2) -> Simplified inverter/3(q2)
  PWM Modulator/1(q1) -> Simplified inverter/2(q1)
  V_ref/1 -> PWM Modulator/2(Compensated error)
  Simplified inverter/1(Vset) -> Vset/1
  Supply voltage/1 -> Simplified inverter/1(Supply voltage), PWM Modulator/1(Supply voltage)

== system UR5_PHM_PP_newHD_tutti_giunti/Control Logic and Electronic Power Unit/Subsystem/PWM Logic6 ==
  V_ref : Inport
  PWM Modulator : Subsystem
  Simplified inverter : Subsystem
  Supply voltage : Constant  Value=U_s
  Vset : Outport
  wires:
  Supply voltage/1 -> PWM Modulator/1(Supply voltage), Simplified inverter/1(Supply voltage)
  Simplified inverter/1(Vset) -> Vset/1
  V_ref/1 -> PWM Modulator/2(Compensated error)
  PWM Modulator/1(q1) -> Simplified inverter/2(q1)
  PWM Modulator/2(q2) -> Simplified inverter/3(q2)

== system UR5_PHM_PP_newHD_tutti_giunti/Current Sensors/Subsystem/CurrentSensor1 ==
  i1 : Inport
  Noise : UniformRandomNumber  Minimum=-var_i(1)  Maximum=var_i(1)  SampleTime=1/50
  "Quantizer " : Quantizer  QuantizationInterval=quant_i(1)
  Sum : Sum  Inputs=|++
  Transfer Fcn (with initial outputs) : simulink_extras/Additional Linear/Transfer Fcn (with initial outputs)  N=[K_i]  D=[tau_i 1]  Y0=I_actual(1,1)  U0=I_actual(1,1)
  "Zero-Order Hold " : ZeroOrderHold  SampleTime=1e-6
  i1FB : Outport
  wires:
  Transfer Fcn (with initial outputs)/1 -> Sum/1
  Sum/1 -> "Zero-Order Hold "/1
  "Zero-Order Hold "/1 -> "Quantizer "/1
  "Quantizer "/1 -> i1FB/1
  Noise/1 -> Sum/2
  i1/1 -> Transfer Fcn (with initial outputs)/1
